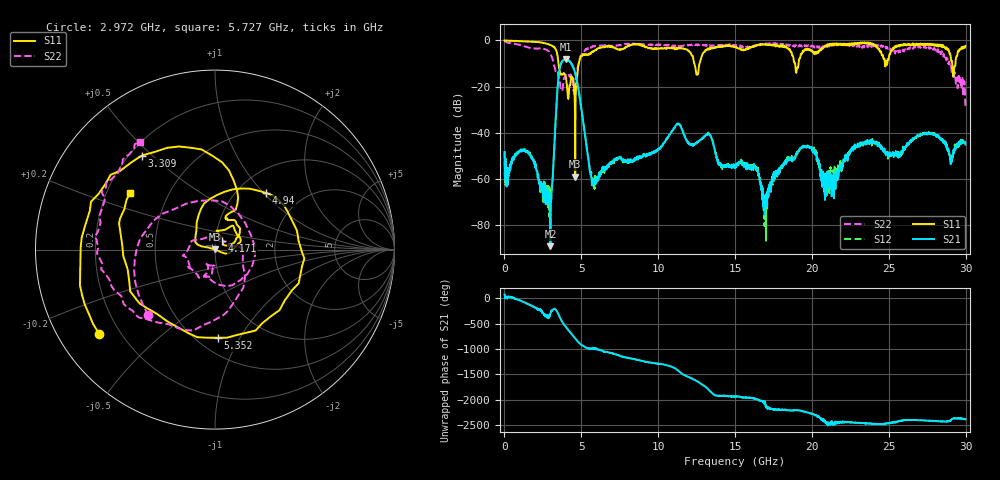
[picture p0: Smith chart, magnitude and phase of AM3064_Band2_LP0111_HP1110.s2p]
# Hz S DB R 50.0
!freq dBS11 angS11 dBS21 angS21 dBS12 angS12 dBS22 angS22
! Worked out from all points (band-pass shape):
!   1600 points, 10 MHz to 29.98 GHz, reference 50 ohm
!   highest |S21| = -8.18 dB at 3.984 GHz (marker M1); lowest = -89.0 dB at 2.99 GHz (marker M2)
!   |S21| within 3 dB of the highest: 3.622 GHz to 4.436 GHz (813.8 MHz wide, 20.2 % of centre)
!   lowest |S11| = -58.9 dB at 4.602 GHz (marker M3), VSWR 1.00, Z = 50.1 + j0.0675 ohm
!   |S11| at or under -10 dB: 3.515 GHz to 4.838 GHz (1.323 GHz wide, 31.7 % of centre); 12.34 GHz to 12.7 GHz (353.9 MHz wide, 2.83 % of centre); 18.9 GHz to 19.13 GHz (228.6 MHz wide, 1.2 % of centre)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
!   |S22| runs from -29.0 to -0.2 dB; largest |S21 - S12| = 0.012
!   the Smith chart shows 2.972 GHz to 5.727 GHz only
!   S11 on the Smith chart (normalised r, x): 2.972 GHz: 0.12, -0.32; 3.309 GHz: 0.25, +0.46; 4.171 GHz: 1.08, +0.10; 4.94 GHz: 1.34, +1.03; 5.352 GHz: 0.63, -0.81; 5.727 GHz: 0.30, +0.28
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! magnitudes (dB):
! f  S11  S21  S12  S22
! 10 MHz  0.0  -48.3  -47.9  -0.2
! 1.472 GHz  -0.5  -48.1  -48.4  -2.9
! 2.972 GHz  -2.0  -75.6  -72.1  -5.7
! 2.99 GHz  -2.0  -89.0  -75.6  -5.9
! 3.309 GHz  -3.6  -37.1  -37.0  -13.0
! 3.59 GHz  -13.0  -12.1  -12.1  -17.0
! 3.984 GHz  -15.6  -8.2  -8.2  -15.0
! 4.171 GHz  -24.3  -8.7  -8.5  -14.7
! 4.602 GHz  -58.9  -14.3  -14.1  -18.7
! 4.94 GHz  -7.4  -26.8  -26.7  -7.0
! 5.015 GHz  -6.8  -30.1  -30.1  -6.3
! 5.352 GHz  -6.2  -46.4  -46.1  -3.6
! 5.727 GHz  -4.9  -62.4  -61.4  -2.7
! 10 GHz  -3.6  -47.1  -47.4  -1.9
! 11.29 GHz  -3.2  -36.2  -36.1  -2.8
! 15 GHz  -2.7  -54.0  -54.6  -2.1
! 16.95 GHz  -1.8  -75.5  -72.1  -1.7
! 19.99 GHz  -4.4  -46.5  -46.7  -2.3
! 21.02 GHz  -1.7  -62.1  -58.8  -2.6
! 25 GHz  -7.9  -49.4  -48.9  -3.1
! 28.31 GHz  -2.3  -42.0  -41.5  -4.7
! 29.98 GHz  -2.4  -45.1  -44.1  -29.0
